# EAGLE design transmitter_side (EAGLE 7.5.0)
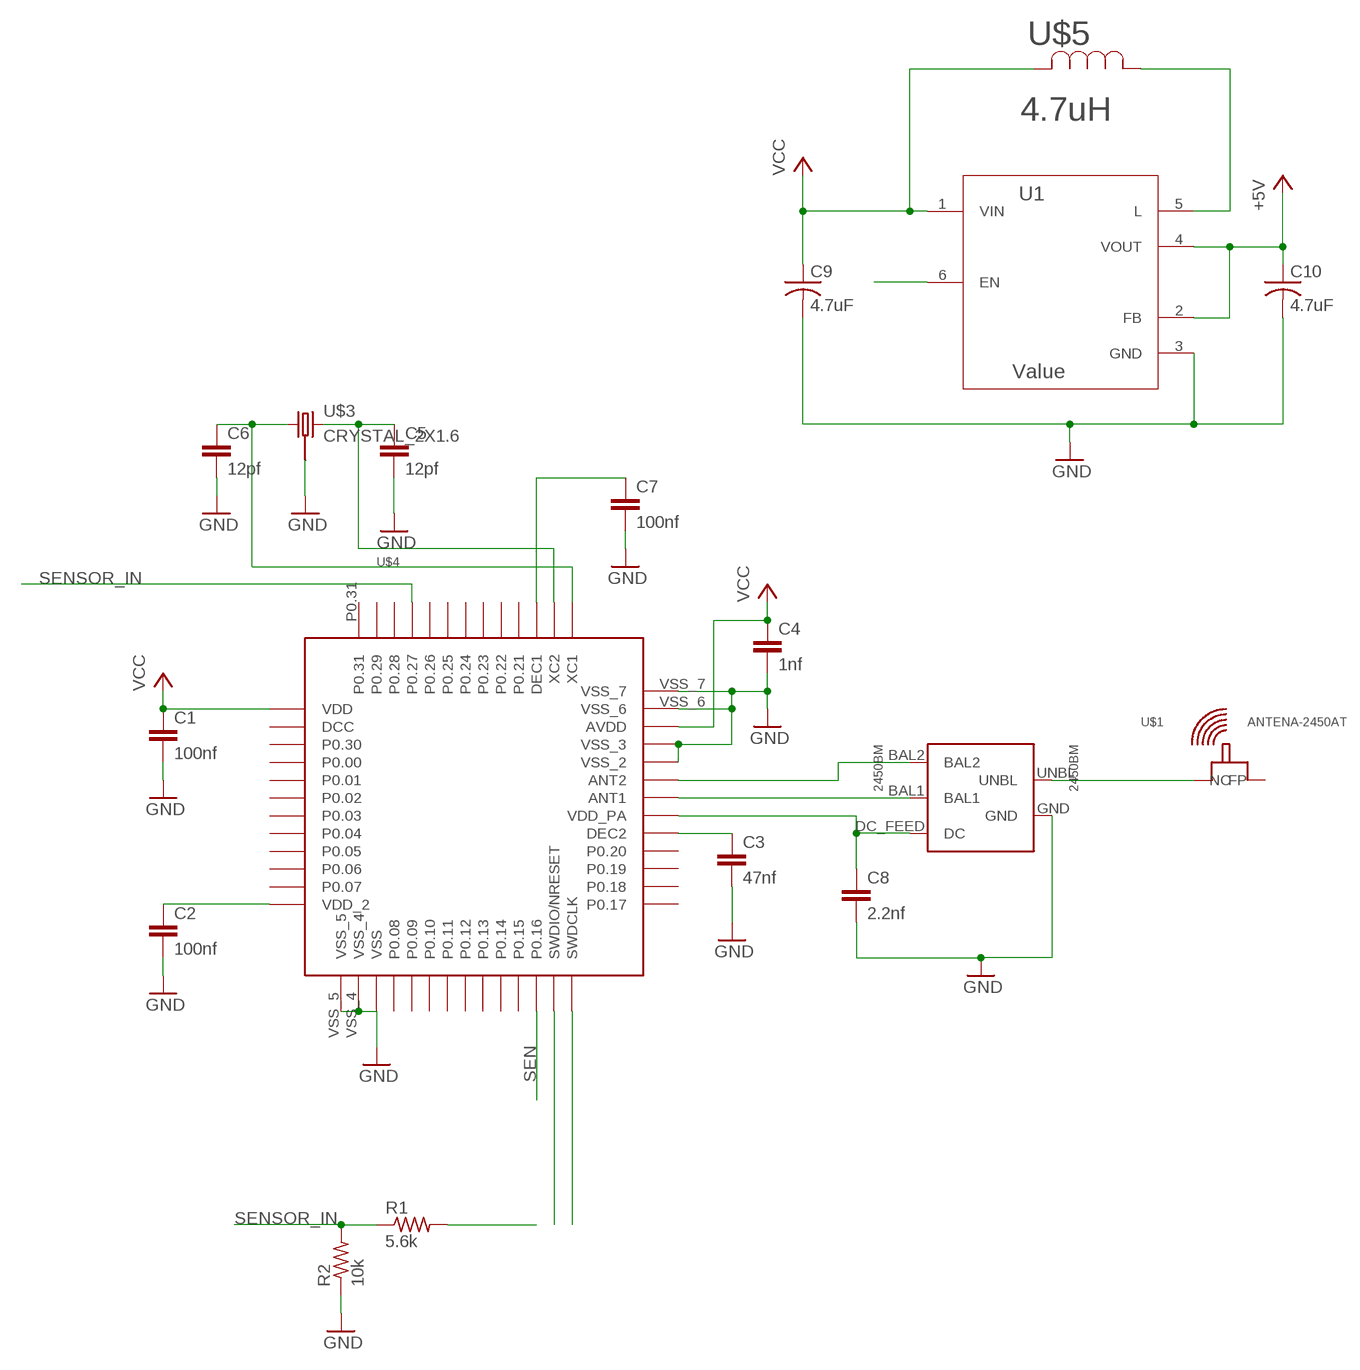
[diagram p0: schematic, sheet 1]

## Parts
2450BM  2450BM  BALUN-2450BM-CEAA  [2450BM08B0003]
C1  100nf  C-EUC0201  [C0201]
C2  100nf  C-EUC0201  [C0201]
C3  47nf  C-EUC0201  [C0201]
C4  1nf  C-EUC0201  [C0201]
C5  12pf  C-EUC0201  [C0201]
C6  12pf  C-EUC0201  [C0201]
C7  100nf  C-EUC0201  [C0201]
C8  2.2nf  C-EUC0201  [C0201]
C9  4.7uF  C-USC0402K  [C0402K]
C10  4.7uF  C-USC0402K  [C0402K]
R1  5.6k  R-US_R0402  [R0402]
R2  10k  R-US_R0402  [R0402]
U1  Value  TPS61222DCKR  [DCK0006A]
U$1  ANTENA-2450AT  [2450AT18B100]
U$3  CRYSTAL_2X1.6  [CRYSTAL_2X1.6MM]
U$4  NRF51822  NRF51822_CEAA  [CEAA_WLCSP]
U$5  4.7uH  L-LQH3NPN4R7MM0L  [IND-4.7UH-LQH3NPN4R7MM0L]

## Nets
+5V: C10.1 U1.2(FB) U1.4(VOUT)
GND: 2450BM.GND C1.2 C2.2 C3.2 C4.2 C5.2 C6.2 C7.2 C8.2 C9.2 C10.2 R2.1 U1.3(GND) U$3.2(GND) U$4.VSS U$4.VSS_2 U$4.VSS_3 U$4.VSS_4 U$4.VSS_5 U$4.VSS_6 U$4.VSS_7
N$1: C6.1 U$3.1 U$4.XC1
N$2: C5.1 U$3.3 U$4.XC2
N$4: C2.1 U$4.VDD_2
N$5: C3.1 U$4.DEC2
N$6: 2450BM.BAL2 U$4.ANT2
N$7: 2450BM.BAL1 U$4.ANT1
N$8: C7.1 U$4.DEC1
N$9: 2450BM.UNBL U$1.FP
N$10: U1.5(L) U$5.1
N$11: U$4.SWDIO(SWDIO/NRESET)
N$12: U$4.SWDCLK
N$13: 2450BM.DC_FEED(DC) C8.1 U$4.VDD_PA
N$15: R1.2
SEN: U1.6(EN) U$4.P0.16
SENSOR_IN: R1.1 R2.2 U$4.P0.27
VCC: C1.1 C4.1 C9.1 U1.1(VIN) U$4.AVDD U$4.VDD U$5.2
Unconnected: U$1.NC U$4.DCC U$4.P0.00 U$4.P0.01 U$4.P0.02 U$4.P0.03 U$4.P0.04 U$4.P0.05 U$4.P0.06 U$4.P0.07 U$4.P0.08 U$4.P0.09 U$4.P0.10 U$4.P0.11 U$4.P0.12 U$4.P0.13 U$4.P0.14 U$4.P0.15 U$4.P0.17 U$4.P0.18 U$4.P0.19 U$4.P0.20 U$4.P0.21 U$4.P0.22 U$4.P0.23 U$4.P0.24 U$4.P0.25 U$4.P0.26 U$4.P0.28 U$4.P0.29 U$4.P0.30 U$4.P0.31

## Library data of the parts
2450BM = NordicSemi:BALUN-2450BM-CEAA
C1-C8 = rcl:C-EU: CAPACITOR, European symbol
C9 C10 = rcl:C-US: CAPACITOR, American symbol
R1 R2 = rcl:R-US_: RESISTOR, American symbol
U1 = texas_extras:TPS61222DCKR; COMPTYPE: IC; MANUFACTURER: Texas Instruments; MOUNTTYPE: SMT; PACKAGEREFERENCE: DCK0006A; PARTNUMBER: TPS61222DCK; PIN_COUNT: 6; REFDES: RefDes; ROHS: Y; TYPE: TYPE
U$1 = NordicSemi:ANTENA-2450AT: General Specifications:
U$3 = custom:CRYSTAL_2X1.6
U$4 = NordicSemi:NRF51822_CEAA
U$5 = custom:L-LQH3NPN4R7MM0L

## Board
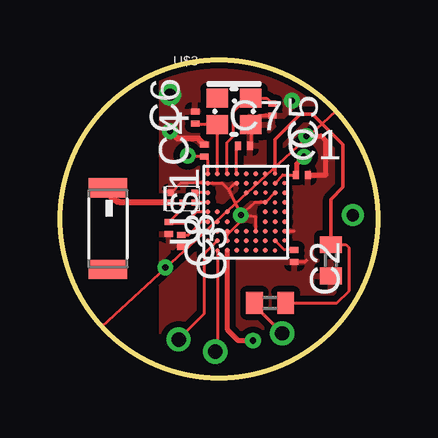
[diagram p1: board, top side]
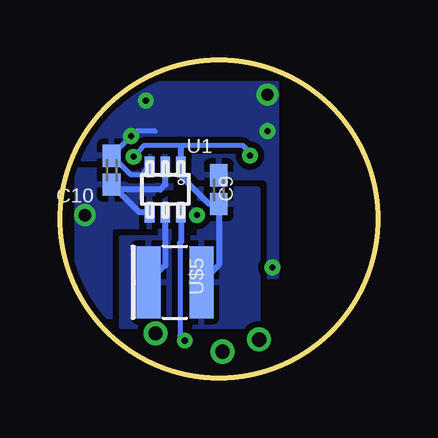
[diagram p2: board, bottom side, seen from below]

Size 13.26 x 13.26 mm. Coordinates in mm from the lower left corner, seen from the top.
Outline: circle at 6.63,6.63 radius 6.63
Copper layers (1*16): Top 0.035mm / dielectric 1.5mm / Bottom 0.035mm
Design rules "default *": minimum track width 5mil, minimum drill 10mil, track to track 5mil, track to pad 5mil, pad to pad 5mil, via to via 5mil, smd to smd 5mil, copper to edge 10mil, drill to drill 8mil, minimum pad ring 10mil, minimum via ring 8mil, stop-mask expansion 4mil, vias tented up to drill 0mil, thermal gap 10mil

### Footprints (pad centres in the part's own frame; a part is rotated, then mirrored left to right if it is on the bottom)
2450BM08B0003 = smd 0.27 x 0.27: BAL1 1.208,0.325; BAL2 1.208,0.725; DC_FEED 0.708,0.325; GND 0.207,0.725; UNBL 0.207,0.325
C0201 = smd 0.25 x 0.35: 1 -0.25,0; 2 0.25,0
C0402K = smd 0.925 x 0.74: 1 -0.6,0; 2 0.6,0
R0402 = smd 0.7 x 0.9: 1 -0.65,0; 2 0.65,0
DCK0006A = smd 0.838 x 0.406: 1 -0.95,0.65; 2 -0.95,0; 3 -0.95,-0.65; 4 0.95,-0.65; 5 0.95,0; 6 0.95,0.65
2450AT18B100 = smd 0.8 x 1.6: FP -1.7,0; NC 1.7,0
CRYSTAL_2X1.6MM = smd 0.9 x 0.8: 1 -0.7,-0.55; 2 0.7,-0.55; 3 0.7,0.55; 4 -0.7,0.55
CEAA_WLCSP = smd 0.2 x 0.2: ANT1 0.15,2.315; ANT2 0.15,2.715; AVDD 0.15,3.515; DEC1 1.35,3.515; DEC2 0.15,1.515; NC 2.15,2.715; NC_2 0.55,1.915; NC_3 0.95,1.915; NC_4 2.55,1.915; NC_5 0.95,1.515; NC_6 2.55,1.515; NC_7 0.95,1.115; NC_8 1.35,1.115; NC_9 1.75,1.115; NC_10 2.55,1.115; P0.00 3.35,2.715; P0.01 3.35,1.915; P0.02 3.35,2.315; P0.03 3.35,1.515; P0.04 2.95,1.515; P0.06 2.95,1.115; P0.07 2.55,0.715; P0.09 2.55,0.315; P0.10 2.15,0.715; P0.11 2.15,0.315; P0.12 1.75,0.315; P0.13 1.75,0.715; P0.14 1.35,0.715; P0.15 1.35,0.315; P0.16 0.95,0.315; P0.17 0.55,1.115; P0.19 0.55,1.515; P0.20 0.15,1.115; P0.21 1.75,3.515; P0.22 1.75,3.115; P0.23 2.15,3.115; P0.24 2.15,3.515; P0.25 1.75,2.715; P0.26 2.55,3.515; P0.28 2.55,3.115; P0.31 2.95,1.915; SWDCLK 0.55,0.715; VDD 2.95,3.115; VDD_2 2.95,0.715; VDD_PA 0.15,1.915; VSS 0.15,3.115; VSS_2 1.35,3.115; VSS_3 2.95,2.715; VSS_4 2.55,2.315; VSS_5 2.15,1.115; VSS_6 3.35,1.115; VSS_7 0.95,0.715; XC1 0.55,3.515; XC2 0.95,3.515 | smd 0.18 x 0.18: DCC 3.35,3.115; P0.05 3.35,0.715; P0.08 2.95,0.315; P0.18 0.15,0.715; P0.27 2.95,3.515; P0.29 2.55,2.715; P0.30 2.95,2.315; SWDIO 0.55,0.315
IND-4.7UH-LQH3NPN4R7MM0L = smd 1 x 3: 1 -1.1,0; 2 1.1,0

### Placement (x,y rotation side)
2450BM  4.42,6.99 0 top
C1  10.08,8.46 0 top
C2  9.78,5.08 270 top
C3  5.05,5.71 270 top
C4  6.02,9.47 90 top
C5  8.86,11.18 270 top
C6  5.64,10.86 90 top
C7  7.67,9.68 0 top
C8  4.55,6.25 270 top
C9  6.63,7.85 90 bottom
C10  11.1,8.66 90 bottom
R1  8.76,3.12 180 top
R2  11.3,4.9 90 top
U1  8.86,7.85 270 bottom
U$1  2.01,6.22 270 top
U$3  7.26,11.11 0 top
U$4  6.02,5 0 top
U$5  8.46,3.99 0 bottom

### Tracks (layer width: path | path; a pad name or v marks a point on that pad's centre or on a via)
+5V  (via drill 0.51 pad 0.51)
  Bottom 0.254: U1.4 9.94,6.9 C10.1 10.89,7.85 9.07,7.85 8.87,8.05 U1.2
  other vias: 12.22,6.78
  pour Bottom (isolate 0.254, rank 2): 8.66,9.27 8.66,7.44 9.27,7.44 9.27,6.02 10.9,6.02 10.9,2.57 12.52,2.57 12.52,8.66 10.49,8.66 10.49,8.25 9.27,8.25 9.27,9.27
GND  (via drill 0.25 pad 0.2, 0.25 pad 0.41, 0.51 pad 0.51)
  Top 0.127: U$4.VSS_5 8.17,6.71 v7.54,6.78 | v7.54,6.78 8.13,7.32 U$4.VSS_4 U$4.VSS_3 | 7.04,7.85 6.77,8.12 U$4.VSS 5.03,8.12 2450BM.GND | 7.04,7.85 v7.54,6.78 | U$4.VSS_2 7.31,8.12 7.04,7.85 | U$3.2 7.96,9.75 C7.2 | U$4.VSS_6 9.78,6.12 | U$4.VSS_7 6.97,5.95 7.64,6.63
  Top 0.152: C5.2 8.33,10.93 U$3.2 | C2.2 10.21,4.83 10.29,4.9
  Top 0.203: C1.2 11.1,8.46 11.1,9.88 10.9,10.08 v10.29,10.08
  Top 0.254: C4.2 5.76,9.98 4.9,9.98 v4.6,10.29
  Bottom 0.203: 9.27,10.29 10.08,10.29 v10.29,10.08 v10.29,10.07 C10.2 10.3,8.46 9.88,8.46 9.54,8.8 U1.3
  Bottom 0.254: 9.47,8.84 U1.3
  other vias: 4.39,4.6 9.68,11.56 4.6,11.81
  pour Top (isolate 0.254, rank 6): 4.19,13.13 4.19,0.74 13.94,0.74 13.94,12.93
  pour Bottom (isolate 0.254, rank 6): 4.19,12.32 12.32,12.32 12.32,4.19 4.19,4.19
  pour Bottom (isolate 0.254, rank 6): 5,7.85 8.46,7.85 8.46,9.47 9.27,9.47 9.27,8.25 10.49,8.25 10.49,8.66 12.52,8.66 12.52,10.9 5,10.9
N$1
  Top 0.127: U$4.XC1 U$3.1 5.68,10.56 C6.1
N$2
  Top 0.127: U$4.XC2 6.97,9.81 7.24,10.08 7.24,11.1 7.8,11.66 U$3.3 8.63,11.66 C5.1
N$4
  Top 0.127: U$4.VDD_2 9.35,5.34 C2.1
N$5
  Top 0.127: U$4.DEC2 5.91,6.52 5.36,5.97 C3.1
N$6
  Top 0.127: U$4.ANT2 2450BM.BAL2
N$7
  Top 0.127: U$4.ANT1 2450BM.BAL1
N$8
  Top 0.127: U$4.DEC1 7.37,9.65 C7.1
N$9
  Top 0.254: 2450BM.UNBL 2.62,7.31 arc-90 U$1.FP
N$10
  Bottom 0.254: U1.5 8.87,4.68 U$5.1
  pour Bottom (isolate 0.254): 8.46,7.44 9.07,7.44 9.07,5.82 10.69,5.82 10.69,2.16 8.46,2.16
N$11  (via drill 0.6)
  Top 0.127: U$4.SWDIO 6.57,1.19 v6.48,1.09
N$12  (via drill 0.6)
  Top 0.127: v4.95,1.6 6.02,2.67 6.01,5.16 6.56,5.71
  Top 0.152: U$4.SWDCLK 6.56,5.71
N$13
  Top 0.127: U$4.VDD_PA 5.7,6.92 5.21,6.43 4.62,6.43 C8.1 5.13,7.08 2450BM.DC_FEED
N$15  (via drill 0.6)
  Top 0.152: R1.2 8.11,3.01 v9.27,1.85
SEN  (via drill 0.25 pad 0.2)
  Top 0.203: v8.05,1.55 7.44,1.55 7.04,1.96 6.97,2.02 U$4.P0.16
  Bottom 0.203: 8.25,5.61 8.25,1.75 v8.05,1.55
  Bottom 0.254: U1.6 8.21,5.65 8.25,5.61
SENSOR_IN
  Top 0.127: R1.1 11.56,3.12 12.07,3.63 12.07,5.41 11.92,5.55 R2.2
  Top 0.152: U$4.P0.27 8.97,9.94 10.03,11 10.54,11 11.81,9.73 11.81,7.95 11.3,7.44 R2.2
VCC  (via drill 0.25 pad 0.2)
  Top 0.127: U$4.VDD 9.3,8.46 C1.1 9.88,8.51 | U$4.AVDD 6.17,9.07 C4.1 5.46,9.22 v5.33,9.27
  Top 0.203: v10.18,9.22 9.88,8.92 9.88,8.51
  Bottom 0.203: v10.18,9.22 9.78,9.68 8.25,9.68 5.61,9.68 5.33,9.4 v5.33,9.27
  Bottom 0.254: U$5.2 6.63,4.72 C9.1 7.05,7.25 8.21,8.42 U1.1 8.21,9.64 8.25,9.68
  pour Bottom (isolate 0.254, rank 3): 8.46,2.16 5,2.16 5,7.85 7.44,7.85 7.44,5.82 8.46,5.82
(copper drawn outside any net)
  shapes: Top area x1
